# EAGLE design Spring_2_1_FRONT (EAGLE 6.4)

## Sheet 1 of 2: Power
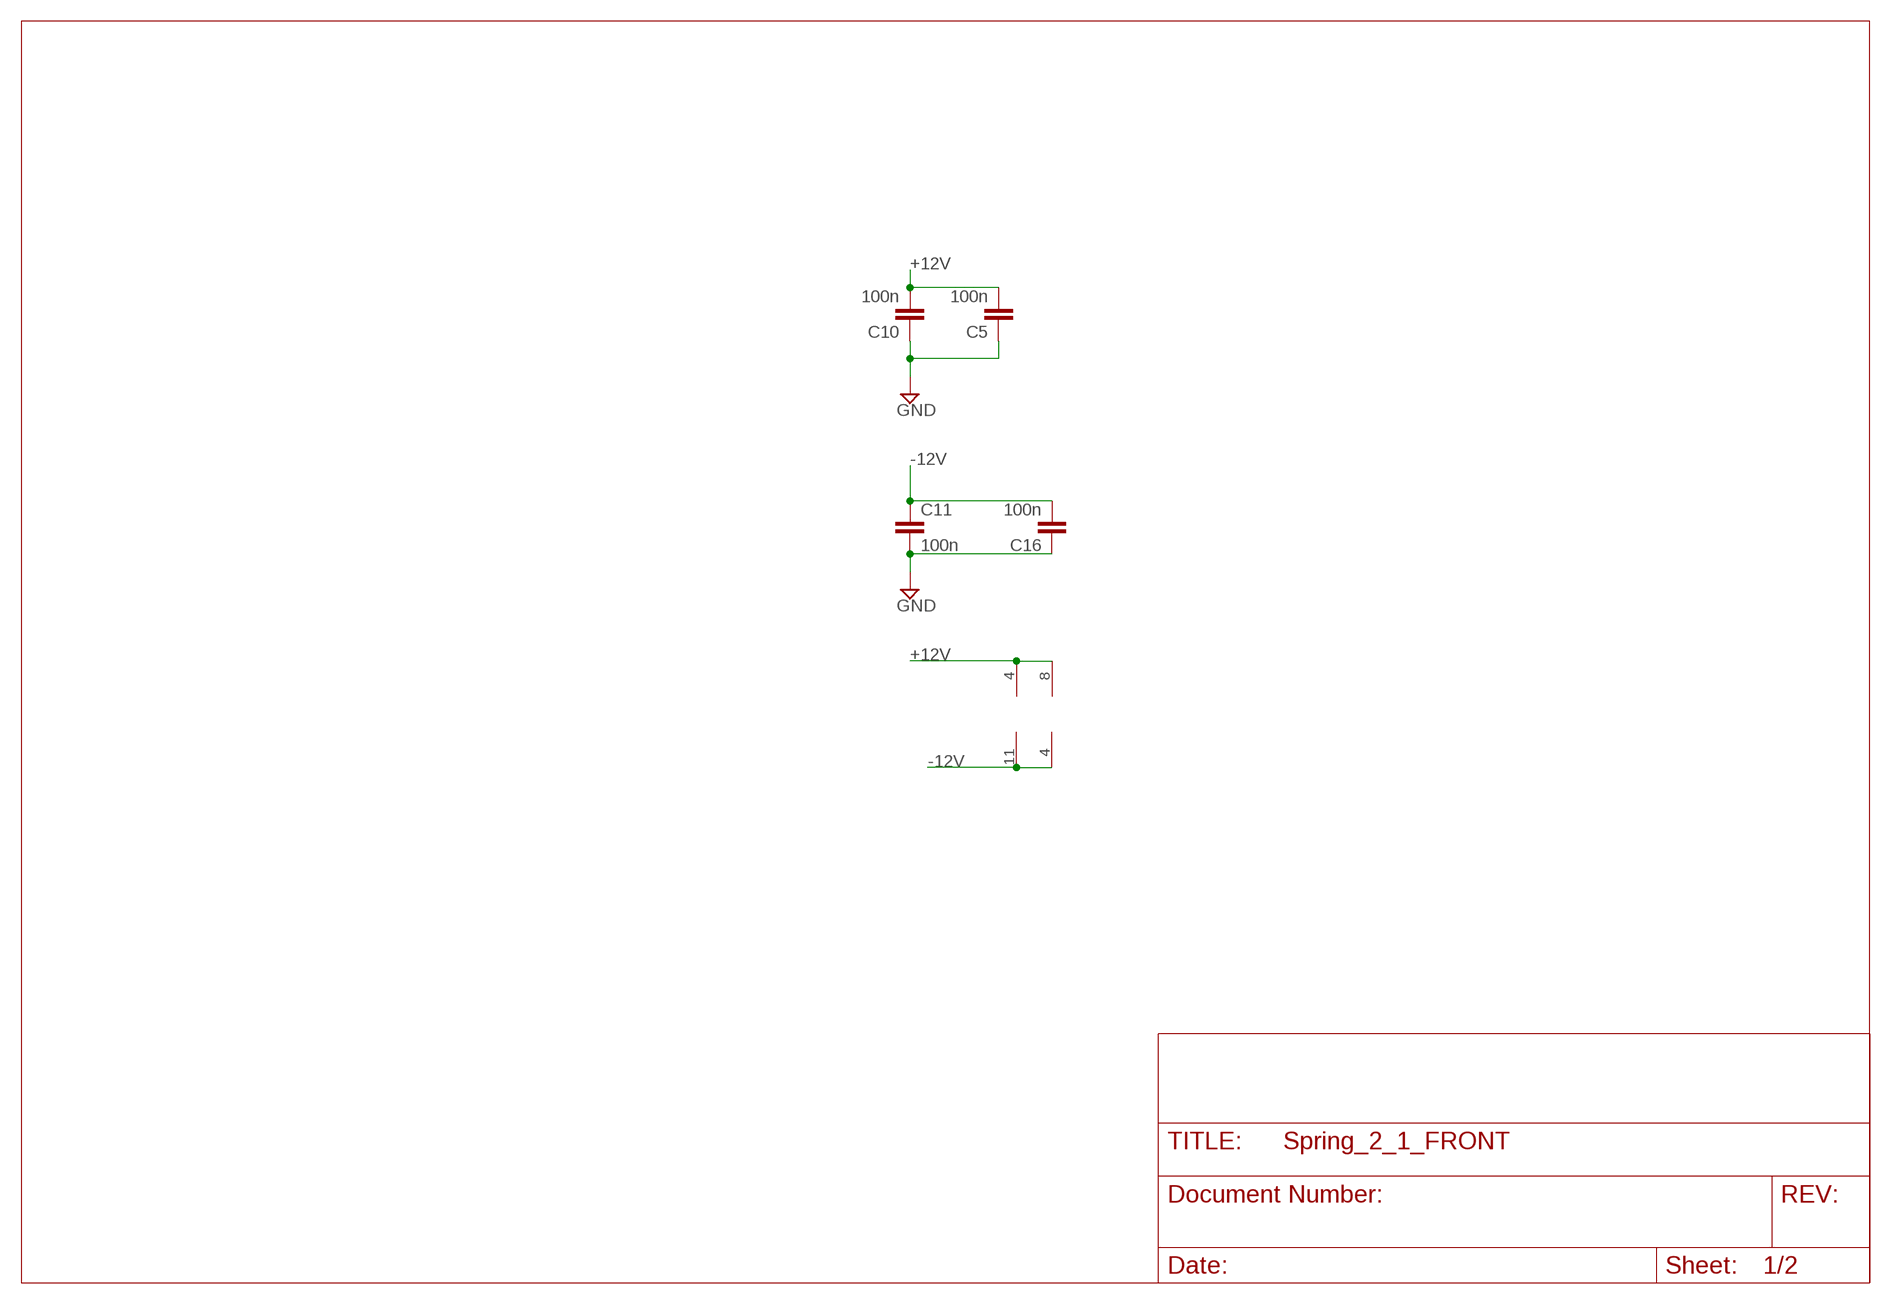
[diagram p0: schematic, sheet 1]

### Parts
C5  100n  C-EU050-024X044  [C050-024X044]
C10  100n  C-EU050-024X044  [C050-024X044]
C11  100n  C-EU050-024X044  [C050-024X044]
C16  100n  C-EU050-024X044  [C050-024X044]
IC1  TL074  TL074P  [DIL14]
IC2_EQ  NE5532  TL072P  [DIL08]

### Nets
+12V [power]: C5.2 C10.2 IC1.4(P:V+) IC2_EQ.8(P:V+) ; also sheet 2
-12V [power]: C11.1 C16.2 IC1.11(P:V-) IC2_EQ.4(P:V-) ; also sheet 2
GND [ground]: C5.1 C10.1 C11.2 C16.1 ; also sheet 2

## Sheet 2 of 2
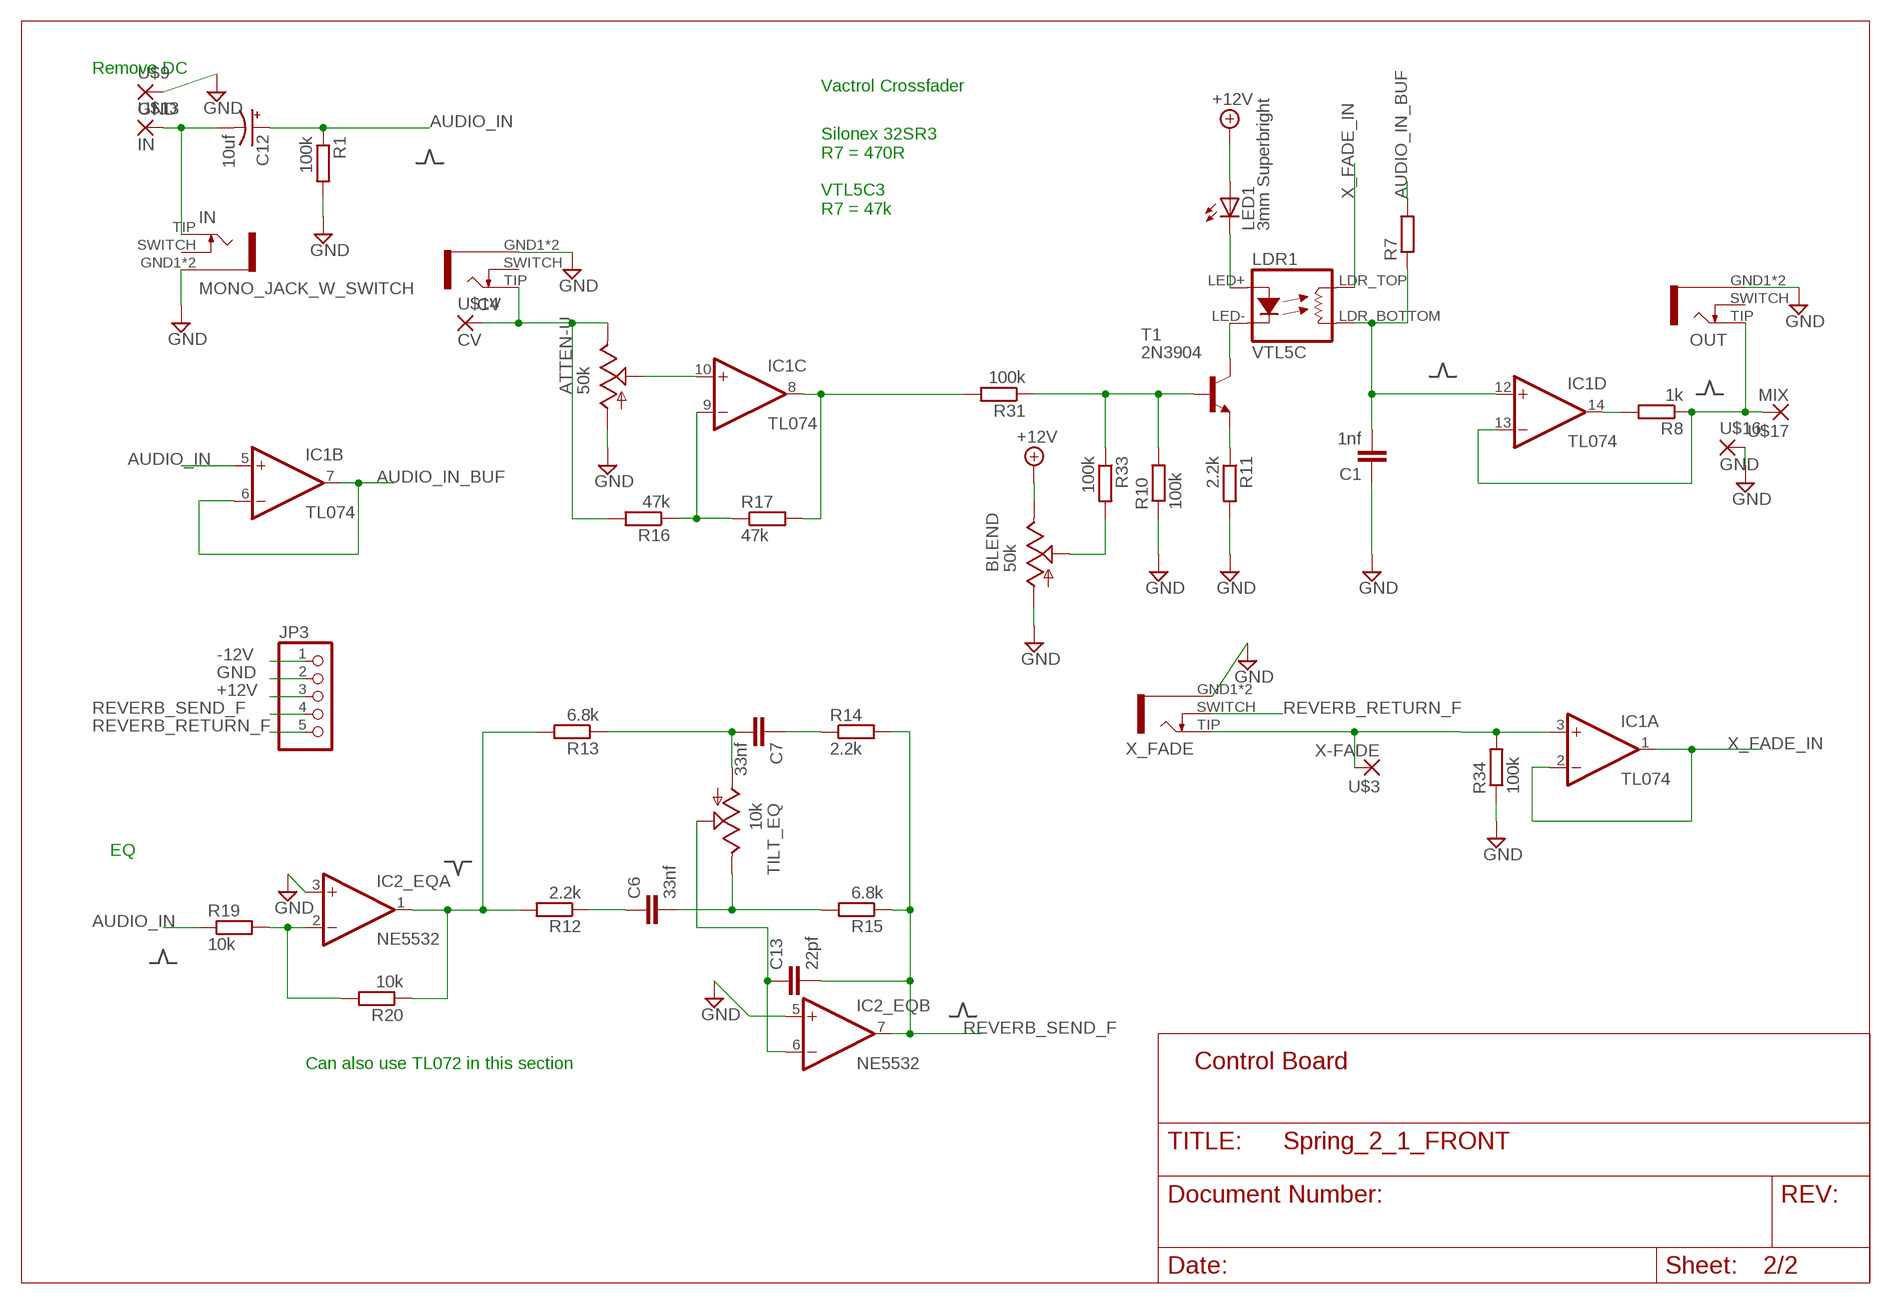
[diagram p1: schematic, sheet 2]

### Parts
ATTEN-U  50k  ALPHA-9MMF2A  [EVUF]
BLEND  50k  ALPHA-9MMF2A  [EVUF]
C1  1nf  C-EU050-024X044  [C050-024X044]
C6  33nf  C-EU050-024X044  [C050-024X044]
C7  33nf  C-EU050-024X044  [C050-024X044]
C12  10uf  050  [050_020]
C13  22pf  050X030_0251  [050X030_025]
CV  MONO_JACK_W_SWITCH  [ERTHENVAR]
IN  MONO_JACK_W_SWITCH  [ERTHENVAR]
JP3  PINHD-1X5  [1X05]
LDR1  VTL5C  VACTROL_COMPACT  [VACTROL_COMPACT]
LED1  3mm Superbright  LED3MM  [LED3MM]
OUT  MONO_JACK_W_SWITCH  [ERTHENVAR]
R1  100k  VERT-RESIST1  [VERT-RESISTOR]
R7  R-EU_STANDARD_RESISTOR  [0207/10]
R8  1k  R-EU_STANDARD_RESISTOR  [0207/10]
R10  100k  R-EU_STANDARD_RESISTOR  [0207/10]
R11  2.2k  R-EU_STANDARD_RESISTOR  [0207/10]
R12  2.2k  R-EU_STANDARD_RESISTOR  [0207/10]
R13  6.8k  R-EU_STANDARD_RESISTOR  [0207/10]
R14  2.2k  R-EU_STANDARD_RESISTOR  [0207/10]
R15  6.8k  R-EU_STANDARD_RESISTOR  [0207/10]
R16  47k  VERT-RESIST1  [VERT-RESISTOR]
R17  47k  VERT-RESIST1  [VERT-RESISTOR]
R19  10k  VERT-RESIST1  [VERT-RESISTOR]
R20  10k  R-EU_STANDARD_RESISTOR  [0207/10]
R31  100k  R-EU_STANDARD_RESISTOR  [0207/10]
R33  100k  R-EU_STANDARD_RESISTOR  [0207/10]
R34  100k  R-EU_STANDARD_RESISTOR  [0207/10]
T1  2N3904  [TO92]
TILT_EQ  10k  ALPHA-9MMF2A  [EVUF]
U$3  X-FADE  LONG_PAD_1  [LONG_PAD_1]
U$9  GND  LONG_PAD_1  [LONG_PAD_1]
U$13  IN  LONG_PAD_1  [LONG_PAD_1]
U$14  CV  LONG_PAD_1  [LONG_PAD_1]
U$16  GND  LONG_PAD_1  [LONG_PAD_1]
U$17  MIX  LONG_PAD_1  [LONG_PAD_1]
X_FADE  MONO_JACK_W_SWITCH  [ERTHENVAR]

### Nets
+12V [power]: BLEND.3(E) JP3.3 LED1.A ; also sheet 1
-12V [power]: JP3.1 ; also sheet 1
AUDIO_IN: C12.+ IC1.5(B:+IN) R1.1 R19.1
AUDIO_IN_BUF: IC1.6(B:-IN) IC1.7(B:OUT) R7.2
GND [ground]: ATTEN-U.1(A) BLEND.1(A) C1.1 CV.GND1(SLEEVE) CV.GND2(SLEEVE) IC2_EQ.3(A:+IN) IC2_EQ.5(B:+IN) IN.GND1(SLEEVE) IN.GND2(SLEEVE) JP3.2 OUT.GND1(SLEEVE) OUT.GND2(SLEEVE) R1.2 R10.1 R11.2 R34.1 U$9.P$1(P) U$16.P$1(P) X_FADE.GND1(SLEEVE) X_FADE.GND2(SLEEVE) ; also sheet 1
MIX_OUT_B: IC1.13(D:-IN) OUT.TIP R8.1 U$17.P$1(P)
N$1: C12.- IN.TIP U$13.P$1(P)
N$3: IC1.3(A:+IN) R34.2 U$3.P$1(P) X_FADE.TIP
N$10: ATTEN-U.3(E) CV.TIP R16.2 U$14.P$1(P)
N$13: C6.1 R12.1
N$14: BLEND.2(S) R33.2
N$15: IC1.14(D:OUT) R8.2
N$16: C6.2 R15.2 TILT_EQ.3(E)
N$17: R11.1 T1.3(E)
N$18: C7.2 R13.1 TILT_EQ.1(A)
N$20: ATTEN-U.2(S) IC1.10(C:+IN)
N$21: C7.1 R14.1
N$22: C13.1 IC2_EQ.6(B:-IN) TILT_EQ.2(S)
N$23: IC1.9(C:-IN) R16.1 R17.1
N$24: IC2_EQ.2(A:-IN) R19.2 R20.2
N$25: IC1.8(C:OUT) R17.2 R31.2
N$26: LDR1.LED+ LED1.K(C)
N$31: IC2_EQ.1(A:OUT) R12.2 R13.2 R20.1
N$36: R10.2 R31.1 R33.1 T1.2(B)
N$37: LDR1.LED- T1.1(C)
REVERB_RETURN_F: JP3.5 X_FADE.SWITCH
REVERB_SEND_F: C13.2 IC2_EQ.7(B:OUT) JP3.4 R14.2 R15.1
SUM: C1.2 IC1.12(D:+IN) LDR1.LDR_BOTTOM(RES2) R7.1
X_FADE_IN: IC1.1(A:OUT) IC1.2(A:-IN) LDR1.LDR_TOP(RES1)
Unconnected: CV.SWITCH IN.SWITCH OUT.SWITCH

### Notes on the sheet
- Remove DC
- Vactrol Crossfader
- Silonex 32SR3 
  R7 = 470R
  
  VTL5C3 
  R7 = 47k
- EQ
- Can also use TL072 in this section | Control Board

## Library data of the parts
ATTEN-U BLEND TILT_EQ = TomW:ALPHA-9MM: 9 mm Square Rotary Potentiometers Source: Panasonic
C1 C5-C7 C10 C11 C16 = TomW:C-EU: CAPACITOR, European symbol
C12 = gm-caps-electro-pol:050: 0.22 - 100uF
C13 = gm-caps-ceramic:050X030_025: 47 - 120pF
CV IN OUT X_FADE = erthenvar:MONO_JACK_W_SWITCH
IC1 = linear:TL074: OP AMP
IC2_EQ = TomW:TL072: OP AMP
JP3 = pinhead:PINHD-1X5: PIN HEADER
LDR1 = TomW:VACTROL_COMPACT
LED1 = TomW:LED: LED
R1 R16 R17 R19 = TomW:VERT-RESIST1: Vertical resistor
R7 R8 R10-R15 R20 R31 R33 R34 = TomW:R-EU_: RESISTOR, European symbol
T1 = transistor:2N3904: NPN TRANSISTOR
U$3 U$9 U$13 U$14 U$16 U$17 = TomW:LONG_PAD_1

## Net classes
0 default: width 0.406 mm
1 power: width 0.61 mm
2 ground: width 0.61 mm

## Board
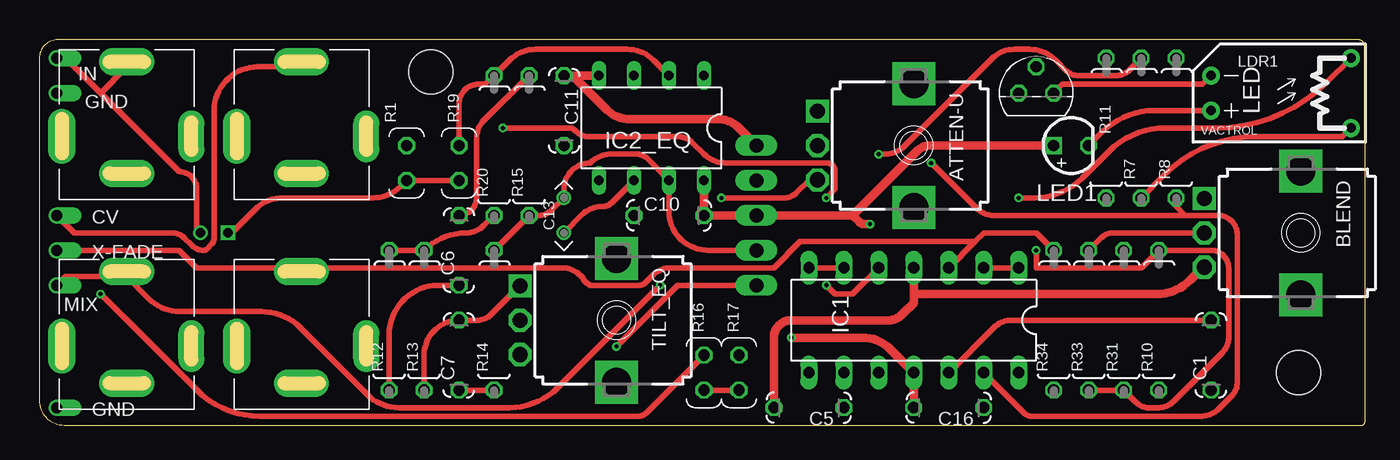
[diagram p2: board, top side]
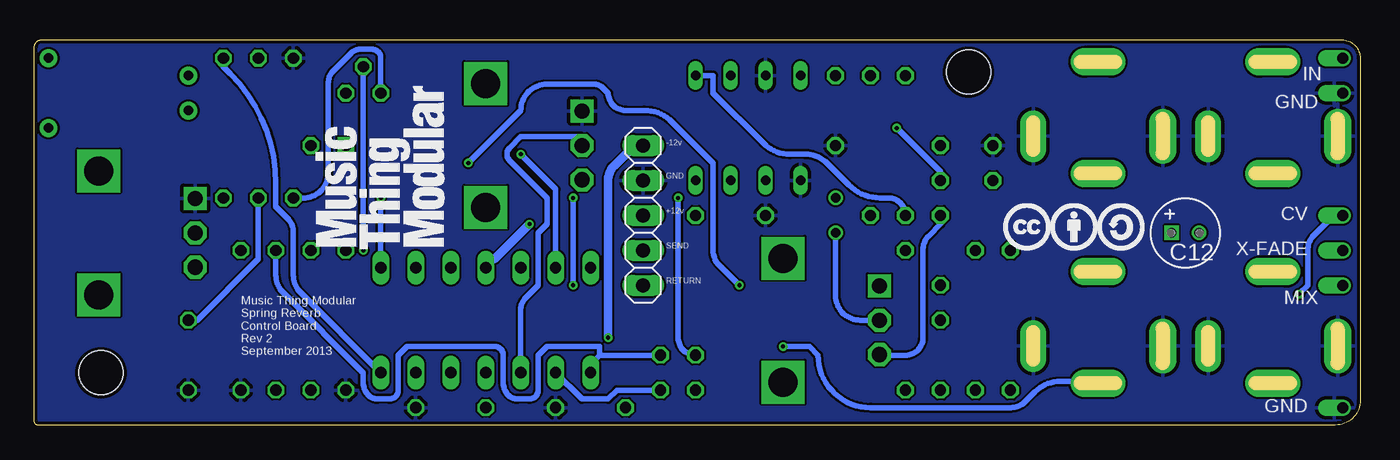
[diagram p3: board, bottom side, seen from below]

Size 96.27 x 28 mm. Coordinates in mm from the lower left corner, seen from the top.
Outline: 1.8,0 96.02,0 arc90 96.27,0.25 96.27,27.48 arc90 95.75,28 1.33,28 arc90 0,26.67 0,1.8 arc90 1.8,0
Copper layers (1*2*15*16): Top 0.035mm / dielectric 0.2mm / Route2 0.0175mm / dielectric 1.1mm / Route15 0.0175mm / dielectric 0.2mm / Bottom 0.035mm
Design rules "SeeedStudio_DRU_no_angle_20130527 *": minimum track width 6mil, minimum drill 12mil, track to track 6mil, track to pad 6mil, pad to pad 6mil, via to via 6mil, smd to smd 0mil, copper to edge 10mil, drill to drill 10mil, minimum pad ring 6mil, minimum via ring 6mil, stop-mask expansion 2mil, vias tented up to drill 25mil, thermal gap 10mil
Holes 3.2 mm at 91.44,3.81 28.45,25.65

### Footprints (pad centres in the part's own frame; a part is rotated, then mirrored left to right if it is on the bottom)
EVUF = drill 1.1 pad 1.676 square: 1 -2.5,-7 | drill 1.1 pad 1.676 octagon: 2 0,-7; 3 2.5,-7 | drill 2.1 pad 2.8 square: M1 4.5,0; M2 -4.5,0
C050-024X044 = drill 0.813 octagon: 1 -2.54,0; 2 2.54,0
050_020 = drill 0.7 square: + -1,0 | drill 0.7: - 1,0
050X030_025 = drill 0.7: 1 -1.27,0; 2 1.27,0
ERTHENVAR = drill 0.5 pad 2 long: GND1 -4.7,-0.6; SWITCH 0,-3.3; TIP 0,4.8 | drill 0.5 pad 1.9 long: GND2 4.7,-0.6
DIL14 = drill 0.813 long: 1 -7.62,-3.81; 2 -5.08,-3.81; 3 -2.54,-3.81; 4 0,-3.81; 5 2.54,-3.81; 6 5.08,-3.81; 7 7.62,-3.81; 8 7.62,3.81; 9 5.08,3.81; 10 2.54,3.81; 11 0,3.81; 12 -2.54,3.81; 13 -5.08,3.81; 14 -7.62,3.81
DIL08 = drill 0.7 long: 1 -3.81,-3.81; 2 -1.27,-3.81; 3 1.27,-3.81; 4 3.81,-3.81; 5 3.81,3.81; 6 1.27,3.81; 7 -1.27,3.81; 8 -3.81,3.81
1X05 = drill 1.016 long: 1 -5.08,0; 2 -2.54,0; 3 0,0; 4 2.54,0; 5 5.08,0
VACTROL_COMPACT = drill 0.7 pad 1.3: LDR_BOTTOM 5.08,-2.54; LDR_TOP 5.08,2.54; LED+ -5.08,-1.27; LED- -5.08,1.27
LED3MM = drill 0.813 square: A -1.27,0 | drill 0.813 octagon: K 1.27,0
VERT-RESISTOR = drill 0.813 octagon: 1 -1.27,0; 2 1.27,0
0207/10 = drill 0.813 octagon: 1 -5.08,0; 2 5.08,0
TO92 = drill 0.813 octagon: 1 1.27,0; 2 0,1.905; 3 -1.27,0
LONG_PAD_1 = drill 0.8 offset: P$1 0,0

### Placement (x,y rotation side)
ATTEN-U  63.5,20.32 270 top
BLEND  91.6,13.97 270 top
C1  85.09,5.08 90 top
C5  55.88,1.27 180 top
C6  30.48,12.7 90 top
C7  30.48,5.08 90 top
C10  45.72,15.24 0 top
C11  38.1,22.86 270 top
C12  12.7,13.97 0 bottom
C13  38.1,15.24 90 top
C16  66.04,1.27 180 top
CV  19.05,21.59 0 top
IC1  63.5,7.62 180 top
IC2_EQ  44.45,21.59 180 top
IN  6.35,21.59 0 top
JP3  52.07,15.24 270 bottom
LDR1  90.17,24.13 0 top
LED1  74.93,20.32 0 top
OUT  6.35,6.35 0 top
R1  26.67,19.05 90 top
R7  80.01,21.59 90 top
R8  82.55,21.59 90 top
R10  81.28,7.62 90 top
R11  77.47,21.59 90 top
R12  25.4,7.62 90 top
R13  27.94,7.62 90 top
R14  33.02,7.62 90 top
R15  35.56,20.32 90 top
R16  48.26,3.81 90 top
R17  50.8,3.81 90 top
R19  30.48,19.05 90 top
R20  33.02,20.32 90 top
R31  78.74,7.62 90 top
R33  76.2,7.62 90 top
R34  73.66,7.62 90 top
T1  72.39,24.13 0 top
TILT_EQ  41.91,7.62 270 top
U$3  1.27,12.7 0 top
U$8  [CC_1CM_SCREENPRINT]  25.91,12.7 0 bottom
U$9  1.27,24.13 0 top
U$10  [MTM_1CM]  66.04,12.7 90 bottom
U$13  1.27,26.67 0 top
U$14  1.27,15.24 0 top
U$16  1.27,1.27 0 top
U$17  1.27,10.16 0 top
X_FADE  19.05,6.35 0 top

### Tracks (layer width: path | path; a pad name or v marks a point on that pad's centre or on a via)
+12V  (via drill 0.3)
  Top 0.61: IC2_EQ.8 C10.2 JP3.3 59.05,15.24 | 59.05,15.24 63.72,19.9 arc-45 64.72,20.32 LED1.A | C5.2 53.34,6.35 arc-90 54.61,7.62 61.7,7.62 arc45 62.6,7.99 63.5,8.89 63.5,9.53 | IC1.4 63.5,9.53 | 63.5,9.53 81.13,9.53 arc45 83.55,10.53 84.45,11.43 BLEND.3 | v60.33,14.61 59.95,14.61 arc-45 59.5,14.79 59.05,15.24
  Bottom 0.61: v60.33,14.61 62.87,12.06 63.5,12.06 IC1.4
-12V  (via drill 0.3)
  Top 0.61: C16.2 IC1.11 61.79,5.52 arc45 59.78,6.35 v54.61,6.35 | C11.1 38.73,25.4 | 38.73,25.4 IC2_EQ.4 | JP3.1 50.75,21.64 arc45 49.33,22.23 42.86,22.23 arc-45 41.24,22.9 38.73,25.4
  Bottom 0.61: v54.61,6.35 54.61,17.83 arc45 54.19,18.83 52.7,20.32 JP3.1
AUDIO_IN  (via drill 0.3)
  Top 0.406: C12.+ 13.97,13.97 15.68,15.68 arc-45 17.69,16.51 24.22,16.51 arc45 26.23,17.34 R1.1 R19.1 | IC1.5 59.05,9.53 57.78,9.53 v57.15,10.16 | v57.15,16.51 57.78,17.14 57.78,18.41 arc90 57.15,19.05 49.84,19.05 arc-45 48.22,19.72 47.41,20.54 arc45 46.4,20.95 39.96,20.95 arc-45 38.95,21.37 38.92,21.4 arc45 38.47,21.59 v33.66,21.59
  Bottom 0.406: v57.15,16.51 v57.15,10.16 | v33.66,21.59 30.48,18.41 R19.1
AUDIO_IN_BUF  (via drill 0.3)
  Top 0.406: IC1.6 IC1.7 | R7.2 79.11,25.77 arc-45 78.21,25.4 75.46,25.4 arc-45 74.56,25.77 73.81,26.52 arc45 71.91,27.3 70.8,27.3 arc45 69.18,26.63 62.79,20.24 arc-45 61.44,19.68 v60.96,19.68
  Bottom 0.406: v60.96,19.68 58.42,17.14 IC1.6
GND
  pour Bottom: -2.54,31.75 99.06,31.75 99.06,-5.08 -2.54,-2.54
MIX_OUT_B  (via drill 0.3)
  Top 0.406: U$17.P$1 1.91,10.79 6.35,10.79 | IC1.13 71.49,0.9 arc45 72.13,0.64 84.3,0.64 arc45 85.65,1.19 86.58,2.12 arc45 87,3.13 87,13.82 arc90 85.58,15.24 83.19,15.24 | 83.19,15.24 82.55,15.88 R8.1 | 6.35,10.79 7.96,9.19 arc45 10.21,8.26 16.1,8.26 arc-45 18.97,7.06 23.84,2.2 arc45 26.08,1.27 34.14,1.27 arc45 37.65,2.72 v45.09,10.16 | 83.19,15.24 69.32,15.24 arc-45 68.05,15.77 v64.77,19.05 | 6.35,10.79 OUT.TIP
  Bottom 0.406: v45.09,10.16 46.57,11.65 arc45 46.99,12.65 46.99,19.05 49.97,22.03 arc-45 51.98,22.86 53.34,22.86 arc90 54.61,24.13 54.98,24.5 arc-45 55.62,24.77 59.05,24.77 arc-90 60.96,22.86 v64.77,19.05
N$1
  Top 0.406: 4.45,24.13 1.91,26.67 U$13.P$1 | 4.45,24.13 10.16,18.41 arc-90 11.43,17.14 11.43,13.97 C12.- | 4.45,24.13 6.35,26.04 IN.TIP
N$3
  Top 0.406: 67.94,13.34 68.58,13.97 72.39,13.97 R34.2 | 67.94,13.34 IC1.3 | 19.05,11.43 37.95,11.43 arc-45 39.29,10.87 39.45,10.72 arc45 40.03,10.16 43.55,10.16 arc45 44,10.35 44.53,10.87 arc-45 45.87,11.43 53.34,11.43 55.24,13.34 67.94,13.34 | U$3.P$1 10.16,12.7 11.43,11.43 19.05,11.43 | 19.05,11.43 X_FADE.TIP
N$10  (via drill 0.3)
  Top 0.406: v49.53,16.51 54.08,16.51 arc45 54.98,16.88 55.88,17.78 ATTEN-U.3 | U$14.P$1 2.54,13.97 9.63,13.97 arc-45 10.53,13.6 11.06,13.07 arc45 11.96,12.7 arc45 12.14,12.78 12.51,13.15 arc45 12.7,13.6 12.7,22.86 arc-90 15.88,26.04 19.05,26.04 CV.TIP | v4.45,9.53 11.42,2.55 arc45 16.04,0.64 43.44,0.64 arc45 44.08,0.9 R16.2
  Bottom 0.406: v49.53,16.51 49.53,6.35 arc-90 R16.2 | v4.45,9.53 3.81,10.16 3.81,12.75 arc45 3.39,13.75 1.91,15.24 U$14.P$1
N$13
  Top 0.406: C6.1 28.99,10.16 arc90 25.4,6.57 R12.1
N$14
  Top 0.406: BLEND.2 78,13.97 arc45 77.1,13.6 R33.2
N$15
  Bottom 0.406: IC1.14 76.94,9.63 arc45 77.47,10.9 77.47,14.02 arc-45 77.89,15.02 78.74,15.88 78.74,17.54 arc-45 82.05,25.54 82.55,26.04 R8.2
N$16
  Top 0.406: C6.2 arc90 31.75,16.51 31.75,20.85 arc-45 32.28,22.12 R15.2
  Bottom 0.406: C6.2 30.48,14.61 31.33,13.75 arc-45 31.75,12.75 31.75,6.35 arc90 33.02,5.08 34.29,5.08 TILT_EQ.3
N$17
  Bottom 0.406: R11.1 76.73,16.51 arc-90 74.93,18.31 74.93,24.87 arc45 74.56,25.77 73.29,27.04 arc45 72.65,27.3 71.75,27.3 arc90 71.12,26.67 T1.3
N$18
  Top 0.406: R13.1 27.94,5.08 arc-90 C7.2 31.8,7.62 arc45 32.8,8.04 34.29,9.53 TILT_EQ.1
N$20
  Bottom 0.406: IC1.10 60.96,8.36 arc45 60.59,9.26 59.69,10.16 59.69,13.97 59.05,14.61 59.05,16.51 61.78,19.24 arc90 61.78,20.13 60.96,20.95 56.52,20.95 56.52,20.32 ATTEN-U.2
N$21
  Top 0.406: R14.1 C7.1
N$22
  Top 0.406: C13.1 39.42,15.29 arc-45 40.84,15.88 40.9,15.88 arc45 41.54,16.14 IC2_EQ.6
  Bottom 0.406: C13.1 38.1,9.42 arc-90 36.3,7.62 TILT_EQ.2
N$23
  Top 0.406: R17.1 R16.1
  Bottom 0.406: IC1.9 56.52,1.91 54.61,1.91 53.98,2.54 R17.1
N$24
  Top 0.406: IC2_EQ.2 44.6,26.52 arc45 42.7,27.3 36.04,27.3 arc45 34.14,26.52 R20.2 32.38,24.77 31.9,24.77 arc90 30.48,23.34 R19.2
N$25
  Bottom 0.406: 55.24,5.08 R17.2 | 55.24,5.08 55.88,4.45 IC1.8 | R31.2 78.74,10.9 arc-45 78.21,9.63 72.39,3.81 72.39,3.07 arc-45 72.02,2.17 arc-45 71.38,1.91 70.48,1.91 arc-90 69.85,2.54 69.85,5.08 69.22,5.71 62.87,5.71 arc90 62.23,5.08 62.23,3.07 arc-45 61.86,2.17 arc-45 61.22,1.91 60.33,1.91 arc-90 59.69,2.54 59.69,5.08 59.05,5.71 55.24,5.71 55.24,5.08
N$26
  Top 0.406: LDR1.LED+ 80.97,22.86 arc45 77.16,21.28 LED1.K
N$31
  Top 0.406: R12.2 R13.2 arc-45 31.01,13.97 arc45 32.28,14.5 R20.1
  Bottom 0.406: IC2_EQ.1 46.99,25.4 46.99,24.13 43.33,20.47 arc-45 41.43,19.68 40.32,19.68 arc45 38.7,19.01 37.12,17.44 arc-45 34.88,16.51 34.29,16.51 arc90 R20.1
N$36  (via drill 0.3)
  Top 0.406: R33.1 R31.1 79.64,1.64 arc45 80.54,1.27 81.33,1.27 arc45 82.33,1.69 85.94,5.3 arc45 86.36,6.3 86.36,11.43 arc90 85.09,12.7 R10.2 80.01,11.43 72.39,11.43 v72.39,12.7
  Bottom 0.406: v72.39,12.7 T1.2
N$37
  Top 0.406: T1.1 74.3,24.77 84.45,24.77 LDR1.LED-
REVERB_RETURN_F  (via drill 0.3)
  Top 0.406: v41.91,5.71 46.35,10.16 JP3.5
  Bottom 0.406: v41.91,5.71 40.01,5.71 39.37,5.08 arc-90 35.56,1.27 25.35,1.27 arc-45 24.35,1.69 23.63,2.41 arc45 21.78,3.17 19.05,3.17 X_FADE.SWITCH
REVERB_SEND_F
  Top 0.406: R14.2 R15.1 36.3,15.24 arc45 37.2,15.61 C13.2 38.1,17.14 arc-90 40.01,19.05 arc-45 41.54,19.68 43.44,19.68 arc-45 44.08,19.42 IC2_EQ.7 45.72,15.54 arc90 48.56,12.7 JP3.4
SUM
  Top 0.406: C1.2 70.59,7.62 arc45 69.32,7.09 IC1.12 | LDR1.LDR_BOTTOM 94.61,20.95 88.34,20.95 arc45 81.71,18.21 R7.1
  Bottom 0.406: R7.1 80.01,12.06 84.45,7.62 C1.2
X_FADE_IN  (via drill 0.3)
  Top 0.406: IC1.1 IC1.2 | LDR1.LDR_TOP 93.5,24.92 arc-45 85.47,21.59 81.8,21.59 arc45 77.66,19.88 75.75,17.96 arc-45 72.24,16.51 v71.12,16.51
  Bottom 0.406: IC1.1 v71.12,16.51

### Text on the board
bPlace: -12v | GND | +12v | SEND | RETURN | Music Thing Modular / Spring Reverb / Control Board / Rev 2 / September 2013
